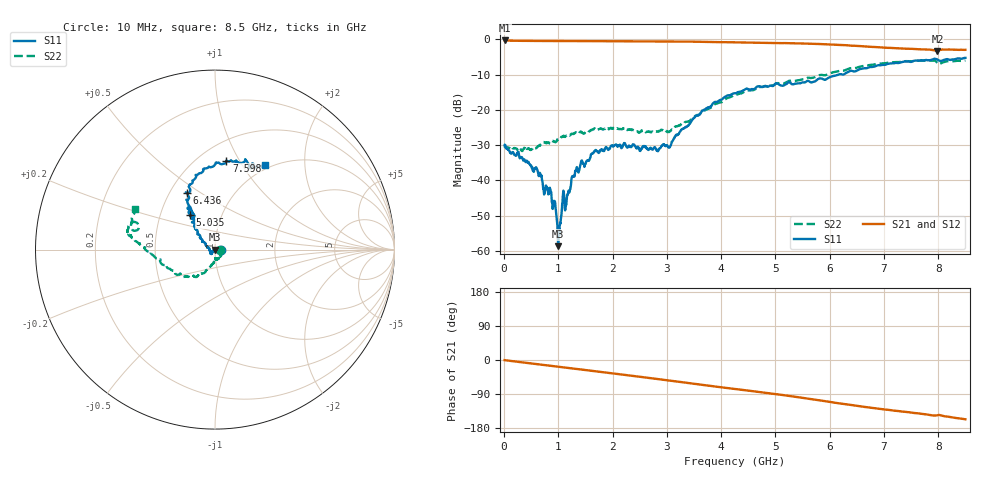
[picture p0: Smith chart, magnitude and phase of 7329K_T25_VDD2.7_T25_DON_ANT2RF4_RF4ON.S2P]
!Agilent Technologies,E5071C,MY46417908,A.11.23
!Date: Mon Aug 31 18:03:24 2020
!Data & Calibration Information:
!Freq	S11:SOLT2(ON)	S21:SOLT2(ON)	S12:SOLT2(ON)	S22:SOLT2(ON)
!PortZ  Port1:50+j0  Port2:50+j0
!Above PortZ is port z conversion or system Z0 setting when saving the data.
!When reading, reference impedance value at option line is always used.
# Hz S dB R 50
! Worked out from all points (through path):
!   1601 points, 10 MHz to 8.5 GHz, reference 50 ohm
!   highest |S21| = -0.33 dB at 10 MHz (marker M1); lowest = -3.3 dB at 7.985 GHz (marker M2)
!   group delay of S21, straight-line fit = 51.6 ps
!   lowest |S11| = -58.6 dB at 997 MHz (marker M3), VSWR 1.00, Z = 50.1 - j0.08 ohm
!   |S11| at or under -10 dB: start of sweep to 6.166 GHz; 6.23328 GHz to 6.251553 GHz (18.27 MHz wide, 0.293 % of centre)
!   |S22| runs from -31.7 to -6.0 dB; largest |S21 - S12| = 0.0064
!   S11 on the Smith chart (normalised r, x): 10 MHz: 1.07, -0.00; 5.035 GHz: 0.71, +0.29; 6.436 GHz: 0.61, +0.44; 7.598 GHz: 0.67, +0.88; 8.5 GHz: 0.95, +1.26
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1e7  -29.96 -1.4  -0.33 -0.3  -0.33 -0.3  -30.67 -5.7
6.308312e8  -38.01 13.9  -0.47 -11.3  -0.47 -11.3  -30.36 -7.9
8.961438e8  -48.09 7.4  -0.49 -16.0  -0.49 -15.9  -28.85 -18.4
9.969625e8  -58.64 -43.1  -0.49 -17.7  -0.49 -17.7  -28.41 -25.9
1.0288e9  -52.61 -76.8  -0.48 -18.3  -0.49 -18.3  -28.19 -27.6
1.076556e9  -46.33 -143.9  -0.50 -19.1  -0.50 -19.1  -27.70 -31.9
1.161456e9  -44.24 -143.0  -0.50 -20.6  -0.50 -20.6  -27.29 -34.8
1.2835e9  -38.73 -138.0  -0.51 -22.8  -0.51 -22.8  -26.79 -42.8
1.426769e9  -34.41 -139.8  -0.52 -25.2  -0.52 -25.3  -26.31 -51.7
1.660244e9  -31.82 -134.7  -0.53 -29.4  -0.53 -29.4  -25.31 -64.9
2.015762e9  -30.26 -132.7  -0.54 -35.6  -0.55 -35.6  -25.24 -76.8
2.843538e9  -31.51 -165.4  -0.60 -50.5  -0.60 -50.5  -26.09 -85.1
3.055788e9  -30.45 172.5  -0.62 -54.4  -0.62 -54.4  -26.04 -86.6
3.681925e9  -19.99 143.1  -0.71 -66.1  -0.71 -66.1  -20.25 -105.3
4.255e9  -15.33 131.5  -0.87 -76.5  -0.87 -76.5  -15.79 -121.2
5.035019e9  -12.53 125.8  -1.08 -90.5  -1.08 -90.4  -12.41 -142.2
5.671769e9  -12.20 122.7  -1.28 -103.4  -1.26 -103.3  -10.95 -162.8
6.435869e9  -9.09 116.2  -1.84 -119.6  -1.86 -119.6  -8.15 178.3
7.088538e9  -6.92 98.5  -2.42 -131.7  -2.44 -131.9  -6.60 172.0
7.597938e9  -6.02 82.7  -2.81 -140.4  -2.82 -140.2  -6.07 168.5
7.985294e9  -5.76 69.1  -3.31 -145.8  -3.33 -145.7  -6.77 161.1
8.5e9  -5.27 59.5  -2.99 -156.5  -3.04 -156.7  -6.01 152.9
